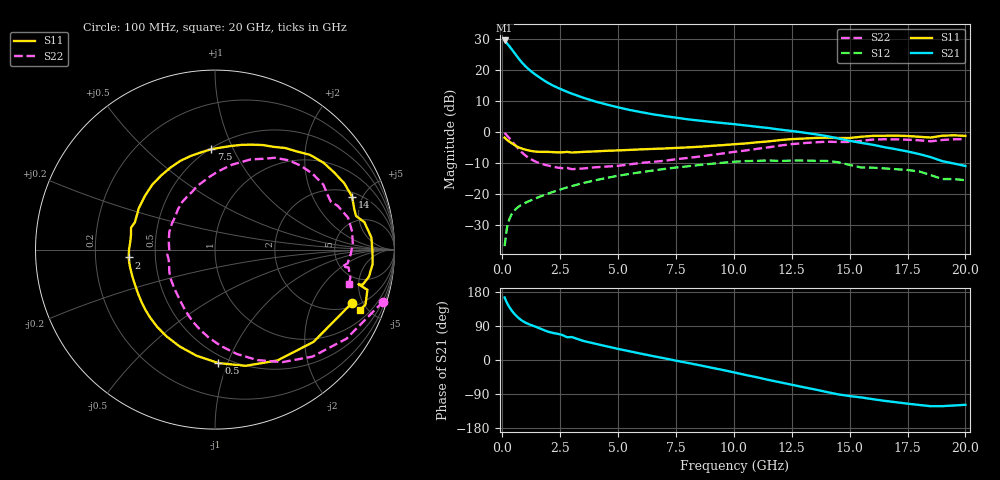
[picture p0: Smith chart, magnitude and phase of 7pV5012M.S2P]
! Infineon Technologies  Discrete & RF Semiconductors
! bfp620
! VCE = 0.50 V,  IC =  12 mA
! Common Emitter S-Parameters:  Sep 2002
# GHz  S  MA  R  50
!  f  S11  S21  S12  S22
! GHz  MAG  ANG  MAG  ANG  MAG  ANG  MAG  ANG
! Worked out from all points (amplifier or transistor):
!   59 points, 100 MHz to 20 GHz, reference 50 ohm
!   highest |S21| = 29.5 dB at 100 MHz (marker M1)
!   |S21| within 3 dB of that: start of sweep to 423.1 MHz
!   unconditionally stable (mu >= 1): 3.75 GHz to 10.1 GHz; 17.12 GHz to end of sweep
!   at 1 GHz: K = 0.57, MSG = 22.0 dB, |S12| = -22.7 dB
!   at 5.5 GHz: K = 1.05, MAG = 8.9 dB, |S12| = -13.4 dB
!   at 20 GHz: K = 1.66, MAG = -2.4 dB, |S12| = -15.4 dB
!   S11 on the Smith chart (normalised r, x): 100 MHz: 2.29, -4.13; 500 MHz: 0.44, -0.93; 2 GHz: 0.35, -0.04; 7.5 GHz: 0.51, +0.82; 14 GHz: 2.31, +4.13; 20 GHz: 1.56, -4.46
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0.1  0.8195 -21.2  29.95 164.9  0.0147 83.0  0.98 -17.2
0.2  0.7522 -43.1  26.9 151.0  0.029 68.2  0.885 -34.1
0.3  0.7089 -60.6  24.27 140.0  0.0397 61.1  0.8063 -47.7
0.4  0.6694 -75.3  21.77 131.0  0.0478 55.9  0.7307 -59.1
0.5  0.6324 -88.3  19.43 123.4  0.054 51.9  0.6588 -69.1
0.6  0.6003 -99.8  17.31 116.8  0.0591 48.8  0.5939 -78.2
0.7  0.5743 -110.1  15.46 111.1  0.0633 46.5  0.538 -86.5
0.8  0.5539 -119.1  13.89 106.2  0.067 44.7  0.4917 -94.0
1  0.5243 -133.3  11.51 98.7  0.0734 42.6  0.4227 -106.5
1.2  0.5036 -144.1  9.859 93.3  0.0793 41.6  0.3756 -116.3
1.4  0.4903 -152.9  8.639 88.7  0.0852 41.0  0.3422 -124.9
2  0.4826 -174.8  6.149 74.3  0.1038 39.0  0.2902 -149.9
2.8  0.4834 165.4  4.468 60.1  0.1296 35.3  0.2667 -174.4
3.5  0.4833 151.4  3.59 50.3  0.1527 30.7  0.2613 170.2
5  0.5104 126.1  2.514 29.3  0.1996 18.8  0.2881 140.3
7  0.5477 98.0  1.82 4.5  0.2567 1.1  0.3472 111.3
7.5  0.5595 92.2  1.715 -1.7  0.2707 -3.8  0.3684 105.5
10.5  0.6596 60.2  1.287 -39.4  0.3435 -36.3  0.5079 73.5
13.5  0.8093 27.2  0.93 -77.7  0.3478 -71.1  0.6885 38.0
14  0.8188 21.1  0.869 -84.3  0.3458 -77.9  0.704 30.9
17  0.8817 -5.3  0.533 -111.4  0.2544 -102.2  0.7682 2.5
20  0.8743 -22.7  0.287 -118.2  0.1694 -114.4  0.7707 -14.2
